(* Logix 5000 DataType export UDT_ISC_InDataConversion; software revision 32.02 *)

TYPE UDT_ISC_InDataConversion :
STRUCT
   ProductsOnBelt : INT;   // Number of products on Intralox belt
   BeltSpeed : INT;   // Belt Speed Input Data from ISC CAM
   LastProductDest : INT;   // Destination of last product inducted input from ISC CAM
   ParameterGroupRead : INT;   // Parameter Group number read - feedback from ISC CAM
   ParameterReadOK : BOOL;   // Parameter read successful feedback from ISC CAM
   ParameterTypeOK : BOOL;   // Parameter type successfull feedback from ISC CAM
   ParameterValueOK : BOOL;   // Parameter value in range successful feedback from ISC CAM
   ParameterWriteOK : BOOL;   // Parameter write successful feedback from ISC CAM
END_STRUCT
END_TYPE
